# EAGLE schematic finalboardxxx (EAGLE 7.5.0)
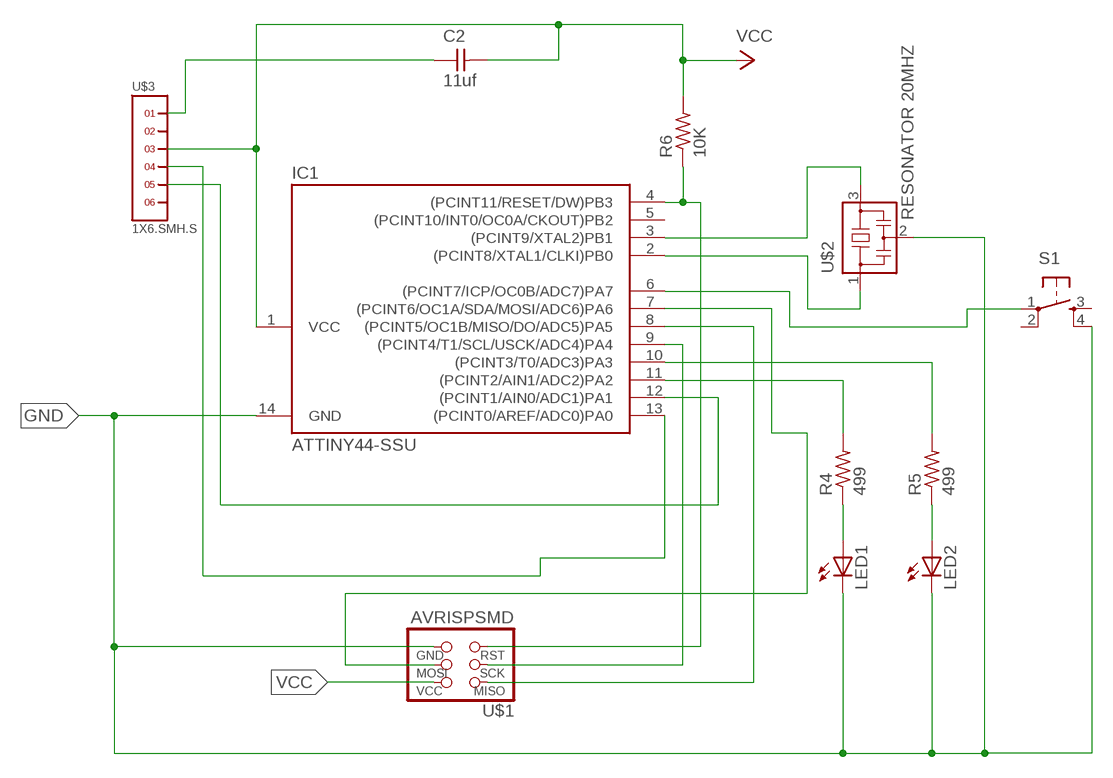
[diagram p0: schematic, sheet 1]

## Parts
C2  11uf  UNPOLARIZED_CAPACITOR1206  [1206]
IC1  ATTINY44-SSU  [SOIC14]
LED1  LED1206  [1206]
LED2  LED1206  [1206]
R4  499  RESISTOR1206  [1206]
R5  499  RESISTOR1206  [1206]
R6  10K  RESISTOR1206  [1206]
S1  6MM_SWITCH6MM_SWITCH  [6MM_SWITCH]
U$1  AVRISPSMD  [2X03SMD]
U$2  RESONATOR 20MHZ  RESONATOR  [EFOBM]
U$3  1X6.SMH.S  [SMH-106-XX-X-S]

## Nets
GND: IC1.14(GND) LED1.2(C) LED2.2(C) S1.4(S1) U$1.6(GND) U$2.2
N$1: IC1.3((PCINT9/XTAL2)PB1) U$2.3
N$2: IC1.2((PCINT8/XTAL1/CLKI)PB0) U$2.1
N$3: C2.1 U$3.1
N$4: IC1.4((PCINT11/RESET/DW)PB3) R6.1 U$1.5(RST)
N$5: IC1.13((PCINT0/AREF/ADC0)PA0) U$3.4
N$6: IC1.12((PCINT1/AIN0/ADC1)PA1) U$3.5
N$7: IC1.9((PCINT4/T1/SCL/USCK/ADC4)PA4) U$1.3(SCK)
N$8: IC1.8((PCINT5/OC1B/MISO/DO/ADC5)PA5) U$1.1(MISO)
N$9: IC1.7((PCINT6/OC1A/SDA/MOSI/ADC6)PA6) U$1.4(MOSI)
N$11: IC1.11((PCINT2/AIN1/ADC2)PA2) R4.2
N$12: LED1.1(A) R4.1
N$13: LED2.1(A) R5.1
N$14: IC1.10((PCINT3/T0/ADC3)PA3) R5.2
N$15: IC1.6((PCINT7/ICP/OC0B/ADC7)PA7) S1.1(P)
VCC: C2.2 IC1.1(VCC) R6.2 U$1.2(VCC) U$3.3
Unconnected: IC1.5((PCINT10/INT0/OC0A/CKOUT)PB2) S1.2(P1) S1.3(S) U$3.2 U$3.6

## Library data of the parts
C2 = FAB_Hello:UNPOLARIZED_CAPACITOR: unpolarized_capacitor
IC1 = fab:ATTINY44
LED1 LED2 = FAB_Hello:LED
R4-R6 = FAB_Hello:RESISTOR
S1 = fab:6MM_SWITCH: OMRON SWITCH
U$1 = FAB_Hello:AVRISP
U$2 = fab:RESONATOR
U$3 = headers(.1in)(samtec):1X6

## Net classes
0 default: width 0.305 mm, drill 0.508 mm, clearance 0.254 mm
